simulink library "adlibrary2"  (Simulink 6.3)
undefined symbols (not defined in the file or in its folder): ad_get_simulink_period, adlibrary2, ADM, blue, Boolean, C, c7c04a0c, CIN, constant, DDRII, gcbh, II, no_bitstream, P, SRAM, SX, VER_STRING_GOES_HERE, white, xlBlockLoadCallback, XP, XRC
libraries: xbsIndex_r4 x299, adlibrary2 x7, adlibrary2_d2sram_0 x5, adlibrary2_ddr_xpi0 x4, adlibrary2_ddr_xpl x3, adlibrary2_xpl32 x1, adlibrary2_xpl64 x1, adlibrary2_zbt64 x1, adlibrary2_zbt4_0 x1, adlibrary2_zbt4_1 x1, adlibrary2_zbt4_2 x1, adlibrary2_zbt4_3 x1
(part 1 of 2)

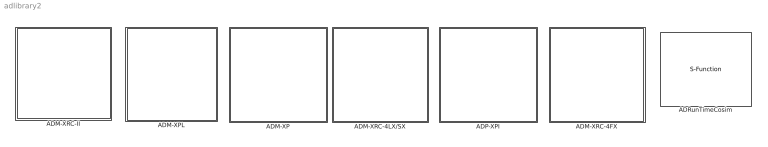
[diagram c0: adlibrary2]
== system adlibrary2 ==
  ADM-XP : Subsystem
  ADM-XPL : Subsystem
  ADM-XRC-4FX : Subsystem  AncestorBlock=adlibrary2/ADM-XRC-4LX//SX
  ADM-XRC-4LX/SX : Subsystem  AncestorBlock=adlibrary2/ADM-XRC-II
  ADM-XRC-II : Subsystem
  ADP-XPI : Subsystem
  ADRunTimeCosim : S-Function  FunctionName=adcosim  Parameters='',index,bitstream,freq,single_step,shared  mask{index=0, bitstream=no_bitstream, freq=50, single_step=off, shared=None}
      mask prompts: index "Card Index"; freq "Clock Frequency"; single_step "Single Step"; shared "Share Access"

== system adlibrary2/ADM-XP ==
  DDR SDRAM 0 : Subsystem  mask{memsize=1}
      mask prompts: memsize "Simulation RAM Size (Mb)"
  DDR SDRAM 1 : Subsystem  mask{memsize=1}
      mask prompts: memsize "Simulation RAM Size (Mb)"
  DDRII SRAM 0 : Subsystem  mask{rate=1}
      mask prompts: rate "Simulink Clock Period"
  DDRII SRAM 1 : Subsystem  AncestorBlock=adlibrary2/ADM-XP/DDRII SRAM 0  mask{rate=1}
      mask prompts: rate "Simulink Clock Period"
  DDRII SRAM 2 : Subsystem  mask{rate=1}
      mask prompts: rate "Simulink Clock Period"
  DDRII SRAM 3 : Subsystem  mask{rate=1}
      mask prompts: rate "Simulink Clock Period"
  XPL 32 Bit Interface : adlibrary2/ADM-XPL/XPL 32 Bit Interface  program='load myprogram.txt'  clock_ratio=1.5  sstep_clk_sel_default=0
  XPL 64 Bit Interface : adlibrary2/ADM-XPL/XPL 64 Bit Interface  program='load myprogram.txt'  clock_ratio=1.5  sstep_clk_sel_default=0

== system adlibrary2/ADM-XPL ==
  DDR SDRAM : Subsystem  mask{memsize=1}
      mask prompts: memsize "Simulation RAM Size (Mb)"
  XPL 32 Bit Interface : Subsystem  mask{program='load myprogram.txt', clock_ratio=1.5, sstep_clk_sel_default=0}
      mask prompts: program "Local Bus Script Program"; clock_ratio "Clock Ratio"
  XPL 64 Bit Interface : Subsystem  mask{program='load myprogram.txt', clock_ratio=1.5, sstep_clk_sel_default=0}
      mask prompts: program "Local Bus Script Program"; clock_ratio "Clock Ratio"
  ZBT SRAM 64 : Subsystem  mask{rate=1}
      mask prompts: rate "Simulink Clock Period"

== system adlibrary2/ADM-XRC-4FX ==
  XPL 32 Bit Interface : adlibrary2/ADM-XPL/XPL 32 Bit Interface  program='load myprogram.txt'  clock_ratio=1.5  sstep_clk_sel_default=0
  XPL 64 Bit Interface : adlibrary2/ADM-XPL/XPL 64 Bit Interface  program='load myprogram.txt'  clock_ratio=1.5  sstep_clk_sel_default=0

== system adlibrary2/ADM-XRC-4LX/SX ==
  PLX 32 Bit Interface : adlibrary2/ADM-XRC-II/PLX 32 Bit Interface  program='load myprogram.txt'  clock_ratio=1.5  sstep_clk_sel_default=0
  ZBT SRAM 0 : Subsystem
  ZBT SRAM 1 : Subsystem
  ZBT SRAM 2 : Subsystem
  ZBT SRAM 3 : Subsystem
  ZBT SRAM 4 : Subsystem
  ZBT SRAM 5 : Subsystem

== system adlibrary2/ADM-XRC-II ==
  PLX 32 Bit Interface : Subsystem  mask{program='load myprogram.txt', clock_ratio=1.5, sstep_clk_sel_default=0}
      mask prompts: program "Local Bus Script Program"; clock_ratio "Clock Ratio"
  "XRM DDR SDRAM " : Subsystem  mask{memsize=1}
      mask prompts: memsize "Simulation RAM Size (Mb)"
  ZBT SRAM 0 : Subsystem  mask{rate=1}
      mask prompts: rate "Simulink Clock Period"
  ZBT SRAM 1 : Subsystem  mask{rate=1}
      mask prompts: rate "Simulink Clock Period"
  ZBT SRAM 2 : Subsystem  mask{rate=1}
      mask prompts: rate "Simulink Clock Period"
  ZBT SRAM 3 : Subsystem  mask{rate=1}
      mask prompts: rate "Simulink Clock Period"
  ZBT SRAM 4 : Subsystem  mask{rate=1}
      mask prompts: rate "Simulink Clock Period"
  ZBT SRAM 5 : Subsystem  mask{rate=1}
      mask prompts: rate "Simulink Clock Period:"

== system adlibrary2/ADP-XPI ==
  DDR SDRAM 0 : Subsystem  mask{memsize=1}
      mask prompts: memsize "Simulation RAM Size (Mb)"
  DDR SDRAM 1 : Subsystem  mask{memsize=1}
      mask prompts: memsize "Simulation RAM Size (Mb)"
  DDR SDRAM 2 : Subsystem  mask{memsize=1}
      mask prompts: memsize "Simulation RAM Size (Mb)"
  DDR SDRAM 3 : Subsystem  mask{memsize=1}
      mask prompts: memsize "Simulation RAM Size (Mb)"
  DDRII SRAM 0 : Subsystem
  XPL 32 Bit Interface : adlibrary2/ADM-XPL/XPL 32 Bit Interface  program='load myprogram.txt'  clock_ratio=1.5  sstep_clk_sel_default=0
  XPL 64 Bit Interface : adlibrary2/ADM-XPL/XPL 64 Bit Interface  program='load myprogram.txt'  clock_ratio=1.5  sstep_clk_sel_default=0

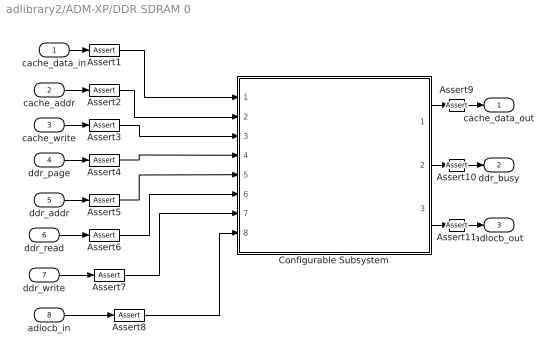
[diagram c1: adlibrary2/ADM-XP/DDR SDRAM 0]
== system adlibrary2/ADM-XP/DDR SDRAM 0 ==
  cache_data_in : Inport
  cache_addr : Inport  Port=2
  cache_write : Inport  Port=3
  ddr_page : Inport  Port=4
  ddr_addr : Inport  Port=5
  ddr_read : Inport  Port=6
  ddr_write : Inport  Port=7
  adlocb_in : Inport  Port=8
  Assert{1..11} (11 alike) : xbsIndex_r4/Assert  assert_type=off  type_source=Explicitly  arith_type="Signed  (2's comp)"  n_bits=16  bin_pt=14  assert_rate=on  rate_source=Explicitly  period=ad_get_simulink_period  output_port=on  block_type=assert
  Configurable Subsystem : Subsystem  Tag=configX  BlockChoice=DDR SDRAM 32bit Simulation  mask{memsize=memsize}
      mask prompts: memsize "Simulation Ram Size (Mb)"
  cache_data_out : Outport
  ddr_busy : Outport  Port=2
  adlocb_out : Outport  Port=3
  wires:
  Configurable Subsystem/3(adlocb_out) -> Assert11/1
  Configurable Subsystem/2(ddr_busy) -> Assert10/1
  Configurable Subsystem/1(cache_data_out) -> Assert9/1
  cache_data_in/1 -> Assert1/1
  cache_addr/1 -> Assert2/1
  cache_write/1 -> Assert3/1
  ddr_page/1 -> Assert4/1
  ddr_addr/1 -> Assert5/1
  ddr_read/1 -> Assert6/1
  ddr_write/1 -> Assert7/1
  adlocb_in/1 -> Assert8/1
  Assert1/1 -> Configurable Subsystem/1(cache_data_in)
  Assert2/1 -> Configurable Subsystem/2(cache_addr)
  Assert3/1 -> Configurable Subsystem/3(cache_write)
  Assert4/1 -> Configurable Subsystem/4(ddr_page)
  Assert5/1 -> Configurable Subsystem/5(ddr_addr)
  Assert6/1 -> Configurable Subsystem/6(ddr_read)
  Assert7/1 -> Configurable Subsystem/7(ddr_write)
  Assert8/1 -> Configurable Subsystem/8(adlocb_in)
  Assert9/1 -> cache_data_out/1
  Assert10/1 -> ddr_busy/1
  Assert11/1 -> adlocb_out/1

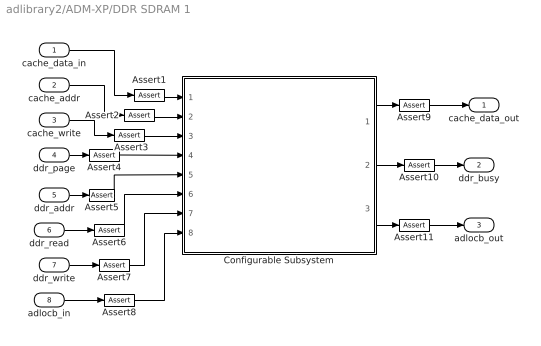
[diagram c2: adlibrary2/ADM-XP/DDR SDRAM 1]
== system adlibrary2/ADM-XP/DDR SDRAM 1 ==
  cache_data_in : Inport
  cache_addr : Inport  Port=2
  cache_write : Inport  Port=3
  ddr_page : Inport  Port=4
  ddr_addr : Inport  Port=5
  ddr_read : Inport  Port=6
  ddr_write : Inport  Port=7
  adlocb_in : Inport  Port=8
  Assert{1..11} (11 alike) : xbsIndex_r4/Assert  assert_type=off  type_source=Explicitly  arith_type="Signed  (2's comp)"  n_bits=16  bin_pt=14  assert_rate=on  rate_source=Explicitly  period=ad_get_simulink_period  output_port=on  block_type=assert
  Configurable Subsystem : Subsystem  Tag=configX  BlockChoice=DDR SDRAM 32bit Simulation  mask{memsize=memsize}
      mask prompts: memsize "Simulation Ram Size (Mb)"
  cache_data_out : Outport
  ddr_busy : Outport  Port=2
  adlocb_out : Outport  Port=3
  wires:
  Configurable Subsystem/3(adlocb_out) -> Assert11/1
  Configurable Subsystem/2(ddr_busy) -> Assert10/1
  Configurable Subsystem/1(cache_data_out) -> Assert9/1
  cache_data_in/1 -> Assert1/1
  cache_addr/1 -> Assert2/1
  cache_write/1 -> Assert3/1
  ddr_page/1 -> Assert4/1
  ddr_addr/1 -> Assert5/1
  ddr_read/1 -> Assert6/1
  ddr_write/1 -> Assert7/1
  adlocb_in/1 -> Assert8/1
  Assert1/1 -> Configurable Subsystem/1(cache_data_in)
  Assert2/1 -> Configurable Subsystem/2(cache_addr)
  Assert3/1 -> Configurable Subsystem/3(cache_write)
  Assert4/1 -> Configurable Subsystem/4(ddr_page)
  Assert5/1 -> Configurable Subsystem/5(ddr_addr)
  Assert6/1 -> Configurable Subsystem/6(ddr_read)
  Assert7/1 -> Configurable Subsystem/7(ddr_write)
  Assert8/1 -> Configurable Subsystem/8(adlocb_in)
  Assert9/1 -> cache_data_out/1
  Assert10/1 -> ddr_busy/1
  Assert11/1 -> adlocb_out/1

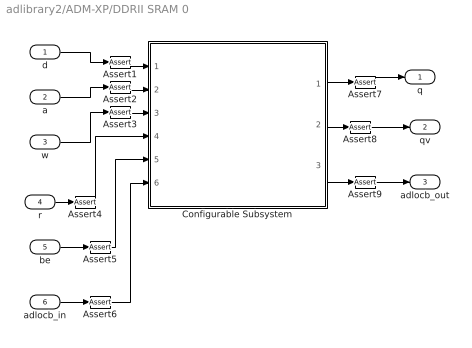
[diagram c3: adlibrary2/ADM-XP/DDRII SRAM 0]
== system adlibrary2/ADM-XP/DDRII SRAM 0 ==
  d : Inport
  a : Inport  Port=2
  w : Inport  Port=3
  r : Inport  Port=4
  be : Inport  Port=5
  adlocb_in : Inport  Port=6
  Assert{1..9} (9 alike) : xbsIndex_r4/Assert  assert_type=off  type_source=Explicitly  arith_type="Signed  (2's comp)"  n_bits=16  bin_pt=14  assert_rate=on  rate_source=Explicitly  period=ad_get_simulink_period  output_port=on  block_type=assert
  Configurable Subsystem : Subsystem  Tag=configX  BlockChoice=DDRII SRAM Simulation
  q : Outport
  qv : Outport  Port=2
  adlocb_out : Outport  Port=3
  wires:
  Configurable Subsystem/1(q) -> Assert7/1
  d/1 -> Assert1/1
  a/1 -> Assert2/1
  w/1 -> Assert3/1
  r/1 -> Assert4/1
  be/1 -> Assert5/1
  adlocb_in/1 -> Assert6/1
  Configurable Subsystem/3(adlocb_out) -> Assert9/1
  Configurable Subsystem/2(qv) -> Assert8/1
  Assert1/1 -> Configurable Subsystem/1(d)
  Assert2/1 -> Configurable Subsystem/2(a)
  Assert3/1 -> Configurable Subsystem/3(w)
  Assert4/1 -> Configurable Subsystem/4(r)
  Assert5/1 -> Configurable Subsystem/5(be)
  Assert6/1 -> Configurable Subsystem/6(adlocb_in)
  Assert7/1 -> q/1
  Assert8/1 -> qv/1
  Assert9/1 -> adlocb_out/1

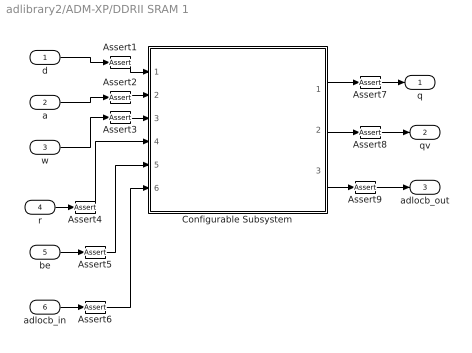
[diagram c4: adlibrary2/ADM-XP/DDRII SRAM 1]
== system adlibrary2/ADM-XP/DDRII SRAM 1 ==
  d : Inport
  a : Inport  Port=2
  w : Inport  Port=3
  r : Inport  Port=4
  be : Inport  Port=5
  adlocb_in : Inport  Port=6
  Assert{1..9} (9 alike) : xbsIndex_r4/Assert  assert_type=off  type_source=Explicitly  arith_type="Signed  (2's comp)"  n_bits=16  bin_pt=14  assert_rate=on  rate_source=Explicitly  period=ad_get_simulink_period  output_port=on  block_type=assert
  Configurable Subsystem : Subsystem  Tag=configX  BlockChoice=DDRII SRAM Simulation
  q : Outport
  qv : Outport  Port=2
  adlocb_out : Outport  Port=3
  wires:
  Configurable Subsystem/1(q) -> Assert7/1
  d/1 -> Assert1/1
  a/1 -> Assert2/1
  w/1 -> Assert3/1
  r/1 -> Assert4/1
  be/1 -> Assert5/1
  adlocb_in/1 -> Assert6/1
  Configurable Subsystem/3(adlocb_out) -> Assert9/1
  Configurable Subsystem/2(qv) -> Assert8/1
  Assert1/1 -> Configurable Subsystem/1(d)
  Assert2/1 -> Configurable Subsystem/2(a)
  Assert3/1 -> Configurable Subsystem/3(w)
  Assert4/1 -> Configurable Subsystem/4(r)
  Assert5/1 -> Configurable Subsystem/5(be)
  Assert6/1 -> Configurable Subsystem/6(adlocb_in)
  Assert7/1 -> q/1
  Assert8/1 -> qv/1
  Assert9/1 -> adlocb_out/1

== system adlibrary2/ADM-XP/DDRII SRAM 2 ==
  d : Inport
  a : Inport  Port=2
  w : Inport  Port=3
  r : Inport  Port=4
  be : Inport  Port=5
  adlocb_in : Inport  Port=6
  Assert{1..9} (9 alike) : xbsIndex_r4/Assert  assert_type=off  type_source=Explicitly  arith_type="Signed  (2's comp)"  n_bits=16  bin_pt=14  assert_rate=on  rate_source=Explicitly  period=ad_get_simulink_period  output_port=on  block_type=assert
  Configurable Subsystem : Subsystem  Tag=configX  BlockChoice=DDRII SRAM Simulation
  q : Outport
  qv : Outport  Port=2
  adlocb_out : Outport  Port=3
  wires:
  Configurable Subsystem/2(qv) -> Assert8/1
  Configurable Subsystem/3(adlocb_out) -> Assert9/1
  adlocb_in/1 -> Assert6/1
  be/1 -> Assert5/1
  r/1 -> Assert4/1
  w/1 -> Assert3/1
  a/1 -> Assert2/1
  d/1 -> Assert1/1
  Configurable Subsystem/1(q) -> Assert7/1
  Assert7/1 -> q/1
  Assert8/1 -> qv/1
  Assert9/1 -> adlocb_out/1
  Assert1/1 -> Configurable Subsystem/1(d)
  Assert2/1 -> Configurable Subsystem/2(a)
  Assert3/1 -> Configurable Subsystem/3(w)
  Assert4/1 -> Configurable Subsystem/4(r)
  Assert5/1 -> Configurable Subsystem/5(be)
  Assert6/1 -> Configurable Subsystem/6(adlocb_in)

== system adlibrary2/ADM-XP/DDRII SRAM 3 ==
  d : Inport
  a : Inport  Port=2
  w : Inport  Port=3
  r : Inport  Port=4
  be : Inport  Port=5
  adlocb_in : Inport  Port=6
  Assert{1..9} (9 alike) : xbsIndex_r4/Assert  assert_type=off  type_source=Explicitly  arith_type="Signed  (2's comp)"  n_bits=16  bin_pt=14  assert_rate=on  rate_source=Explicitly  period=ad_get_simulink_period  output_port=on  block_type=assert
  Configurable Subsystem : Subsystem  Tag=configX  BlockChoice=DDRII SRAM Simulation
  q : Outport
  qv : Outport  Port=2
  adlocb_out : Outport  Port=3
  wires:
  Configurable Subsystem/2(qv) -> Assert8/1
  Configurable Subsystem/3(adlocb_out) -> Assert9/1
  adlocb_in/1 -> Assert6/1
  be/1 -> Assert5/1
  r/1 -> Assert4/1
  w/1 -> Assert3/1
  a/1 -> Assert2/1
  d/1 -> Assert1/1
  Configurable Subsystem/1(q) -> Assert7/1
  Assert1/1 -> Configurable Subsystem/1(d)
  Assert2/1 -> Configurable Subsystem/2(a)
  Assert3/1 -> Configurable Subsystem/3(w)
  Assert4/1 -> Configurable Subsystem/4(r)
  Assert5/1 -> Configurable Subsystem/5(be)
  Assert6/1 -> Configurable Subsystem/6(adlocb_in)
  Assert7/1 -> q/1
  Assert8/1 -> qv/1
  Assert9/1 -> adlocb_out/1

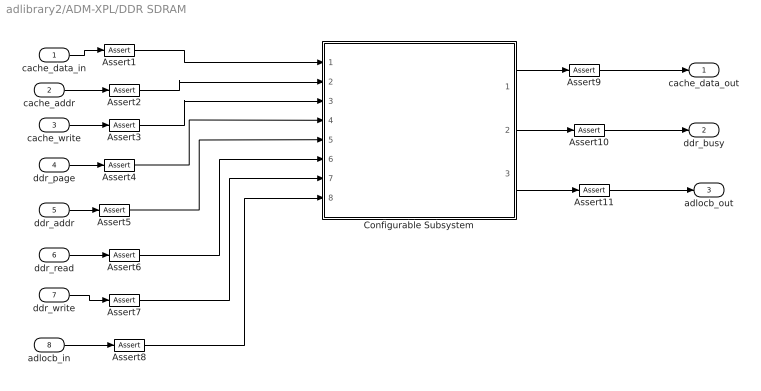
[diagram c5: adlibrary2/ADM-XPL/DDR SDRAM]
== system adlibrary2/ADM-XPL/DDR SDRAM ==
  cache_data_in : Inport
  cache_addr : Inport  Port=2
  cache_write : Inport  Port=3
  ddr_page : Inport  Port=4
  ddr_addr : Inport  Port=5
  ddr_read : Inport  Port=6
  ddr_write : Inport  Port=7
  adlocb_in : Inport  Port=8
  Assert{1..11} (11 alike) : xbsIndex_r4/Assert  assert_type=off  type_source=Explicitly  arith_type="Signed  (2's comp)"  n_bits=16  bin_pt=14  assert_rate=on  rate_source=Explicitly  period=ad_get_simulink_period  output_port=on  block_type=assert
  Configurable Subsystem : Subsystem  Tag=configX  BlockChoice=DDR SDRAM 32bit Simulation  mask{memsize=memsize}
      mask prompts: memsize "Simulation Ram Size (Mb)"
  cache_data_out : Outport
  ddr_busy : Outport  Port=2
  adlocb_out : Outport  Port=3
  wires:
  cache_data_in/1 -> Assert1/1
  cache_addr/1 -> Assert2/1
  cache_write/1 -> Assert3/1
  ddr_page/1 -> Assert4/1
  ddr_addr/1 -> Assert5/1
  ddr_read/1 -> Assert6/1
  ddr_write/1 -> Assert7/1
  adlocb_in/1 -> Assert8/1
  Configurable Subsystem/1(cache_data_out) -> Assert9/1
  Configurable Subsystem/2(ddr_busy) -> Assert10/1
  Configurable Subsystem/3(adlocb_out) -> Assert11/1
  Assert1/1 -> Configurable Subsystem/1(cache_data_in)
  Assert2/1 -> Configurable Subsystem/2(cache_addr)
  Assert3/1 -> Configurable Subsystem/3(cache_write)
  Assert4/1 -> Configurable Subsystem/4(ddr_page)
  Assert5/1 -> Configurable Subsystem/5(ddr_addr)
  Assert6/1 -> Configurable Subsystem/6(ddr_read)
  Assert7/1 -> Configurable Subsystem/7(ddr_write)
  Assert8/1 -> Configurable Subsystem/8(adlocb_in)
  Assert9/1 -> cache_data_out/1
  Assert10/1 -> ddr_busy/1
  Assert11/1 -> adlocb_out/1

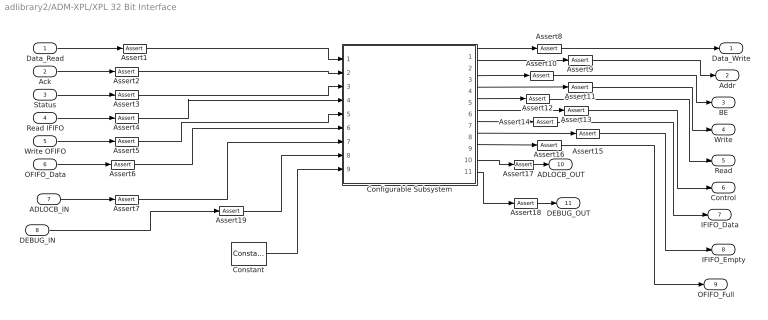
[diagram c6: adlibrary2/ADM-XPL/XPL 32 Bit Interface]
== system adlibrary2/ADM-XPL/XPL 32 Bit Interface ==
  Data_Read : Inport
  Ack : Inport  Port=2
  Status : Inport  Port=3
  Read IFIFO : Inport  Port=4
  Write OFIFO : Inport  Port=5
  OFIFO_Data : Inport  Port=6
  ADLOCB_IN : Inport  Port=7
  DEBUG_IN : Inport  Port=8
  Assert{1..19} (19 alike) : xbsIndex_r4/Assert  assert_type=off  type_source=Explicitly  arith_type="Signed  (2's comp)"  n_bits=16  bin_pt=14  assert_rate=on  rate_source=Explicitly  period=ad_get_simulink_period  output_port=on  block_type=assert
  Configurable Subsystem : Subsystem  Tag=configX  BlockChoice=XPL 32Bit Simulation  mask{program=program, clock_ratio=clock_ratio}
      mask prompts: program "Local Bus Script Program"; clock_ratio "Clock Ratio"
  Constant : xbsIndex_r4/Constant  arith_type=Boolean  const=sstep_clk_sel_default  n_bits=16  bin_pt=14  explicit_period=on  period=ad_get_simulink_period  equ=P=C  opselect=C  inp2=PCIN>>17  opr=+  inp1=P  carry=CIN  dbl_ovrd=off  block_type=constant
  Data_Write : Outport
  Addr : Outport  Port=2
  BE : Outport  Port=3
  Write : Outport  Port=4
  Read : Outport  Port=5
  Control : Outport  Port=6
  IFIFO_Data : Outport  Port=7
  IFIFO_Empty : Outport  Port=8
  OFIFO_Full : Outport  Port=9
  ADLOCB_OUT : Outport  Port=10
  DEBUG_OUT : Outport  Port=11
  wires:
  Status/1 -> Assert3/1
  Ack/1 -> Assert2/1
  Data_Read/1 -> Assert1/1
  Configurable Subsystem/9(OFIFO_Full) -> Assert16/1
  Configurable Subsystem/8(IFIFO_Empty) -> Assert15/1
  Configurable Subsystem/7(IFIFO_Data) -> Assert14/1
  Configurable Subsystem/6(Control) -> Assert13/1
  Configurable Subsystem/5(Read) -> Assert12/1
  Configurable Subsystem/4(Write) -> Assert11/1
  Configurable Subsystem/3(BE) -> Assert10/1
  Configurable Subsystem/1(Data_Write) -> Assert8/1
  Configurable Subsystem/2(Addr) -> Assert9/1
  Read IFIFO/1 -> Assert4/1
  Write OFIFO/1 -> Assert5/1
  OFIFO_Data/1 -> Assert6/1
  ADLOCB_IN/1 -> Assert7/1
  Configurable Subsystem/10(ADLOCB_OUT) -> Assert17/1
  Assert1/1 -> Configurable Subsystem/1(Data_Read)
  Assert2/1 -> Configurable Subsystem/2(Ack)
  Assert3/1 -> Configurable Subsystem/3(Status)
  Assert4/1 -> Configurable Subsystem/4(Read IFIFO)
  Assert8/1 -> Data_Write/1
  Assert9/1 -> Addr/1
  Assert10/1 -> BE/1
  Assert11/1 -> Write/1
  Assert12/1 -> Read/1
  Assert13/1 -> Control/1
  Assert14/1 -> IFIFO_Data/1
  Assert15/1 -> IFIFO_Empty/1
  Assert16/1 -> OFIFO_Full/1
  Assert17/1 -> ADLOCB_OUT/1
  Assert5/1 -> Configurable Subsystem/5(Write OFIFO)
  Assert6/1 -> Configurable Subsystem/6(OFIFO_Data)
  Assert7/1 -> Configurable Subsystem/7(ADLOCB_IN)
  DEBUG_IN/1 -> Assert19/1
  Assert19/1 -> Configurable Subsystem/8(DEBUG_IN)
  Assert18/1 -> DEBUG_OUT/1
  Configurable Subsystem/11(DEBUG_OUT) -> Assert18/1
  Constant/1 -> Configurable Subsystem/9(sstep_clk_sel_default)

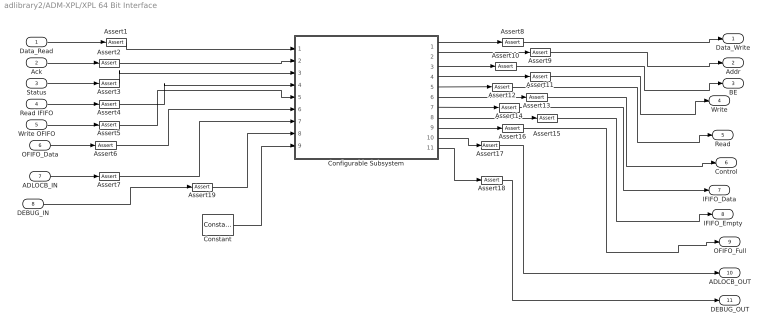
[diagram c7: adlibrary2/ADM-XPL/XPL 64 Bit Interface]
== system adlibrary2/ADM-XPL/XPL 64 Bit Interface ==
  Data_Read : Inport
  Ack : Inport  Port=2
  Status : Inport  Port=3
  Read IFIFO : Inport  Port=4
  Write OFIFO : Inport  Port=5
  OFIFO_Data : Inport  Port=6
  ADLOCB_IN : Inport  Port=7
  DEBUG_IN : Inport  Port=8
  Assert{1..19} (19 alike) : xbsIndex_r4/Assert  assert_type=off  type_source=Explicitly  arith_type="Signed  (2's comp)"  n_bits=16  bin_pt=14  assert_rate=on  rate_source=Explicitly  period=ad_get_simulink_period  output_port=on  block_type=assert
  Configurable Subsystem : Subsystem  Tag=configX  BlockChoice=XPL 64Bit Simulation  mask{program=program, clock_ratio=clock_ratio}
      mask prompts: program "Local Bus Script Program"; clock_ratio "Clock Ratio"
  Constant : xbsIndex_r4/Constant  arith_type=Boolean  const=sstep_clk_sel_default  n_bits=16  bin_pt=14  explicit_period=on  period=ad_get_simulink_period  equ=P=C  opselect=C  inp2=PCIN>>17  opr=+  inp1=P  carry=CIN  dbl_ovrd=off  block_type=constant
  Data_Write : Outport
  Addr : Outport  Port=2
  BE : Outport  Port=3
  Write : Outport  Port=4
  Read : Outport  Port=5
  Control : Outport  Port=6
  IFIFO_Data : Outport  Port=7
  IFIFO_Empty : Outport  Port=8
  OFIFO_Full : Outport  Port=9
  ADLOCB_OUT : Outport  Port=10
  DEBUG_OUT : Outport  Port=11
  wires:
  Status/1 -> Assert3/1
  Ack/1 -> Assert2/1
  Data_Read/1 -> Assert1/1
  Read IFIFO/1 -> Assert4/1
  Write OFIFO/1 -> Assert5/1
  OFIFO_Data/1 -> Assert6/1
  ADLOCB_IN/1 -> Assert7/1
  Assert1/1 -> Configurable Subsystem/1(Data_Read)
  Assert2/1 -> Configurable Subsystem/2(Ack)
  Assert3/1 -> Configurable Subsystem/3(Status)
  Assert4/1 -> Configurable Subsystem/4(Read IFIFO)
  Assert5/1 -> Configurable Subsystem/5(Write OFIFO)
  Assert6/1 -> Configurable Subsystem/6(OFIFO_Data)
  Assert7/1 -> Configurable Subsystem/7(ADLOCB_IN)
  DEBUG_IN/1 -> Assert19/1
  Assert19/1 -> Configurable Subsystem/8(DEBUG_IN)
  Constant/1 -> Configurable Subsystem/9(sstep_clk_sel_default)
  Configurable Subsystem/9(OFIFO_Full) -> Assert16/1
  Configurable Subsystem/8(IFIFO_Empty) -> Assert15/1
  Configurable Subsystem/7(IFIFO_Data) -> Assert14/1
  Configurable Subsystem/6(Control) -> Assert13/1
  Configurable Subsystem/5(Read) -> Assert12/1
  Configurable Subsystem/4(Write) -> Assert11/1
  Configurable Subsystem/3(BE) -> Assert10/1
  Configurable Subsystem/1(Data_Write) -> Assert8/1
  Configurable Subsystem/2(Addr) -> Assert9/1
  Configurable Subsystem/10(ADLOCB_OUT) -> Assert17/1
  Assert8/1 -> Data_Write/1
  Assert9/1 -> Addr/1
  Assert10/1 -> BE/1
  Assert11/1 -> Write/1
  Assert12/1 -> Read/1
  Assert13/1 -> Control/1
  Assert14/1 -> IFIFO_Data/1
  Assert15/1 -> IFIFO_Empty/1
  Assert16/1 -> OFIFO_Full/1
  Assert17/1 -> ADLOCB_OUT/1
  Assert18/1 -> DEBUG_OUT/1
  Configurable Subsystem/11(DEBUG_OUT) -> Assert18/1

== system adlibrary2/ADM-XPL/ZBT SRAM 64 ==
  d : Inport
  a : Inport  Port=2
  w : Inport  Port=3
  r : Inport  Port=4
  be : Inport  Port=5
  adlocb_in : Inport  Port=6
  Assert{1..9} (9 alike) : xbsIndex_r4/Assert  assert_type=off  type_source=Explicitly  arith_type="Signed  (2's comp)"  n_bits=16  bin_pt=14  assert_rate=on  rate_source=Explicitly  period=ad_get_simulink_period  output_port=on  block_type=assert
  Configurable Subsystem : Subsystem  Tag=configX  BlockChoice=ZBT SRAM 64bit Simulation
  q : Outport
  qv : Outport  Port=2
  adlocb_out : Outport  Port=3
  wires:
  d/1 -> Assert1/1
  a/1 -> Assert2/1
  w/1 -> Assert3/1
  r/1 -> Assert4/1
  be/1 -> Assert5/1
  adlocb_in/1 -> Assert6/1
  Configurable Subsystem/1(q) -> Assert7/1
  Configurable Subsystem/2(qv) -> Assert8/1
  Configurable Subsystem/3(adlocb_out) -> Assert9/1
  Assert1/1 -> Configurable Subsystem/1(d)
  Assert2/1 -> Configurable Subsystem/2(a)
  Assert3/1 -> Configurable Subsystem/3(w)
  Assert4/1 -> Configurable Subsystem/4(r)
  Assert5/1 -> Configurable Subsystem/5(be)
  Assert6/1 -> Configurable Subsystem/6(adlocb_in)
  Assert7/1 -> q/1
  Assert8/1 -> qv/1
  Assert9/1 -> adlocb_out/1

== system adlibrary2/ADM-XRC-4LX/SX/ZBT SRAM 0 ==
  d : Inport
  a : Inport  Port=2
  w : Inport  Port=3
  r : Inport  Port=4
  be : Inport  Port=5
  adlocb_in : Inport  Port=6
  Assert{1..9} (9 alike) : xbsIndex_r4/Assert  assert_type=off  type_source=Explicitly  arith_type="Signed  (2's comp)"  n_bits=16  bin_pt=14  assert_rate=on  rate_source=Explicitly  period=ad_get_simulink_period  output_port=on  block_type=assert
  Configurable Subsystem : Subsystem  Tag=configX  BlockChoice=ZBT SRAM 32Bit Simulation
  q : Outport
  qv : Outport  Port=2
  adlocb_out : Outport  Port=3
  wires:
  Configurable Subsystem/3(adlocb_out) -> Assert9/1
  Configurable Subsystem/2(qv) -> Assert8/1
  Configurable Subsystem/1(q) -> Assert7/1
  adlocb_in/1 -> Assert6/1
  be/1 -> Assert5/1
  r/1 -> Assert4/1
  w/1 -> Assert3/1
  a/1 -> Assert2/1
  d/1 -> Assert1/1
  Assert1/1 -> Configurable Subsystem/1(d)
  Assert2/1 -> Configurable Subsystem/2(a)
  Assert3/1 -> Configurable Subsystem/3(w)
  Assert4/1 -> Configurable Subsystem/4(r)
  Assert5/1 -> Configurable Subsystem/5(be)
  Assert6/1 -> Configurable Subsystem/6(adlocb_in)
  Assert7/1 -> q/1
  Assert8/1 -> qv/1
  Assert9/1 -> adlocb_out/1

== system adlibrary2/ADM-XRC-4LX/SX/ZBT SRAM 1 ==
  d : Inport
  a : Inport  Port=2
  w : Inport  Port=3
  r : Inport  Port=4
  be : Inport  Port=5
  adlocb_in : Inport  Port=6
  Assert{1..9} (9 alike) : xbsIndex_r4/Assert  assert_type=off  type_source=Explicitly  arith_type="Signed  (2's comp)"  n_bits=16  bin_pt=14  assert_rate=on  rate_source=Explicitly  period=ad_get_simulink_period  output_port=on  block_type=assert
  Configurable Subsystem : Subsystem  Tag=configX  BlockChoice=ZBT SRAM 32Bit Simulation
  q : Outport
  qv : Outport  Port=2
  adlocb_out : Outport  Port=3
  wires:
  d/1 -> Assert1/1
  a/1 -> Assert2/1
  w/1 -> Assert3/1
  r/1 -> Assert4/1
  be/1 -> Assert5/1
  adlocb_in/1 -> Assert6/1
  Configurable Subsystem/1(q) -> Assert7/1
  Configurable Subsystem/2(qv) -> Assert8/1
  Configurable Subsystem/3(adlocb_out) -> Assert9/1
  Assert1/1 -> Configurable Subsystem/1(d)
  Assert2/1 -> Configurable Subsystem/2(a)
  Assert3/1 -> Configurable Subsystem/3(w)
  Assert4/1 -> Configurable Subsystem/4(r)
  Assert5/1 -> Configurable Subsystem/5(be)
  Assert6/1 -> Configurable Subsystem/6(adlocb_in)
  Assert7/1 -> q/1
  Assert8/1 -> qv/1
  Assert9/1 -> adlocb_out/1

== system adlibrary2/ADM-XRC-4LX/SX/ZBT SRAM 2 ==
  d : Inport
  a : Inport  Port=2
  w : Inport  Port=3
  r : Inport  Port=4
  be : Inport  Port=5
  adlocb_in : Inport  Port=6
  Assert{1..9} (9 alike) : xbsIndex_r4/Assert  assert_type=off  type_source=Explicitly  arith_type="Signed  (2's comp)"  n_bits=16  bin_pt=14  assert_rate=on  rate_source=Explicitly  period=ad_get_simulink_period  output_port=on  block_type=assert
  Configurable Subsystem : Subsystem  Tag=configX  BlockChoice=ZBT SRAM 32Bit Simulation
  q : Outport
  qv : Outport  Port=2
  adlocb_out : Outport  Port=3
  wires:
  d/1 -> Assert1/1
  a/1 -> Assert2/1
  w/1 -> Assert3/1
  r/1 -> Assert4/1
  be/1 -> Assert5/1
  adlocb_in/1 -> Assert6/1
  Configurable Subsystem/1(q) -> Assert8/1
  Configurable Subsystem/2(qv) -> Assert9/1
  Configurable Subsystem/3(adlocb_out) -> Assert7/1
  Assert1/1 -> Configurable Subsystem/1(d)
  Assert2/1 -> Configurable Subsystem/2(a)
  Assert3/1 -> Configurable Subsystem/3(w)
  Assert4/1 -> Configurable Subsystem/4(r)
  Assert5/1 -> Configurable Subsystem/5(be)
  Assert6/1 -> Configurable Subsystem/6(adlocb_in)
  Assert7/1 -> adlocb_out/1
  Assert8/1 -> q/1
  Assert9/1 -> qv/1

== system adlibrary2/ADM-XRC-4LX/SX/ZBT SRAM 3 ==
  d : Inport
  a : Inport  Port=2
  w : Inport  Port=3
  r : Inport  Port=4
  be : Inport  Port=5
  adlocb_in : Inport  Port=6
  Assert{1..9} (9 alike) : xbsIndex_r4/Assert  assert_type=off  type_source=Explicitly  arith_type="Signed  (2's comp)"  n_bits=16  bin_pt=14  assert_rate=on  rate_source=Explicitly  period=ad_get_simulink_period  output_port=on  block_type=assert
  Configurable Subsystem : Subsystem  Tag=configX  BlockChoice=ZBT SRAM 32Bit Simulation
  q : Outport
  qv : Outport  Port=2
  adlocb_out : Outport  Port=3
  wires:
  d/1 -> Assert1/1
  a/1 -> Assert2/1
  w/1 -> Assert3/1
  r/1 -> Assert4/1
  be/1 -> Assert5/1
  adlocb_in/1 -> Assert6/1
  Configurable Subsystem/1(q) -> Assert7/1
  Configurable Subsystem/2(qv) -> Assert8/1
  Configurable Subsystem/3(adlocb_out) -> Assert9/1
  Assert1/1 -> Configurable Subsystem/1(d)
  Assert2/1 -> Configurable Subsystem/2(a)
  Assert3/1 -> Configurable Subsystem/3(w)
  Assert4/1 -> Configurable Subsystem/4(r)
  Assert5/1 -> Configurable Subsystem/5(be)
  Assert6/1 -> Configurable Subsystem/6(adlocb_in)
  Assert7/1 -> q/1
  Assert8/1 -> qv/1
  Assert9/1 -> adlocb_out/1

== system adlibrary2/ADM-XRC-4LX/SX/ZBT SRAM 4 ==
  d : Inport
  a : Inport  Port=2
  w : Inport  Port=3
  r : Inport  Port=4
  be : Inport  Port=5
  adlocb_in : Inport  Port=6
  Assert{1..9} (9 alike) : xbsIndex_r4/Assert  assert_type=off  type_source=Explicitly  arith_type="Signed  (2's comp)"  n_bits=16  bin_pt=14  assert_rate=on  rate_source=Explicitly  period=ad_get_simulink_period  output_port=on  block_type=assert
  Configurable Subsystem : Subsystem  Tag=configX  BlockChoice=ZBT SRAM 32Bit Simulation
  q : Outport
  qv : Outport  Port=2
  adlocb_out : Outport  Port=3
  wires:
  d/1 -> Assert1/1
  a/1 -> Assert2/1
  w/1 -> Assert3/1
  r/1 -> Assert4/1
  be/1 -> Assert5/1
  adlocb_in/1 -> Assert6/1
  Configurable Subsystem/1(q) -> Assert7/1
  Configurable Subsystem/2(qv) -> Assert8/1
  Configurable Subsystem/3(adlocb_out) -> Assert9/1
  Assert1/1 -> Configurable Subsystem/1(d)
  Assert2/1 -> Configurable Subsystem/2(a)
  Assert3/1 -> Configurable Subsystem/3(w)
  Assert4/1 -> Configurable Subsystem/4(r)
  Assert5/1 -> Configurable Subsystem/5(be)
  Assert6/1 -> Configurable Subsystem/6(adlocb_in)
  Assert7/1 -> q/1
  Assert8/1 -> qv/1
  Assert9/1 -> adlocb_out/1

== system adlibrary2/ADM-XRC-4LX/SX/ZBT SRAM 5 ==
  d : Inport
  a : Inport  Port=2
  w : Inport  Port=3
  r : Inport  Port=4
  be : Inport  Port=5
  adlocb_in : Inport  Port=6
  Assert{1..9} (9 alike) : xbsIndex_r4/Assert  assert_type=off  type_source=Explicitly  arith_type="Signed  (2's comp)"  n_bits=16  bin_pt=14  assert_rate=on  rate_source=Explicitly  period=ad_get_simulink_period  output_port=on  block_type=assert
  Configurable Subsystem : Subsystem  Tag=configX  BlockChoice=ZBT SRAM 32Bit Simulation
  q : Outport
  qv : Outport  Port=2
  adlocb_out : Outport  Port=3
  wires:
  d/1 -> Assert1/1
  a/1 -> Assert2/1
  w/1 -> Assert3/1
  r/1 -> Assert4/1
  be/1 -> Assert5/1
  adlocb_in/1 -> Assert6/1
  Configurable Subsystem/1(q) -> Assert7/1
  Configurable Subsystem/2(qv) -> Assert8/1
  Configurable Subsystem/3(adlocb_out) -> Assert9/1
  Assert1/1 -> Configurable Subsystem/1(d)
  Assert2/1 -> Configurable Subsystem/2(a)
  Assert3/1 -> Configurable Subsystem/3(w)
  Assert4/1 -> Configurable Subsystem/4(r)
  Assert5/1 -> Configurable Subsystem/5(be)
  Assert6/1 -> Configurable Subsystem/6(adlocb_in)
  Assert7/1 -> q/1
  Assert8/1 -> qv/1
  Assert9/1 -> adlocb_out/1

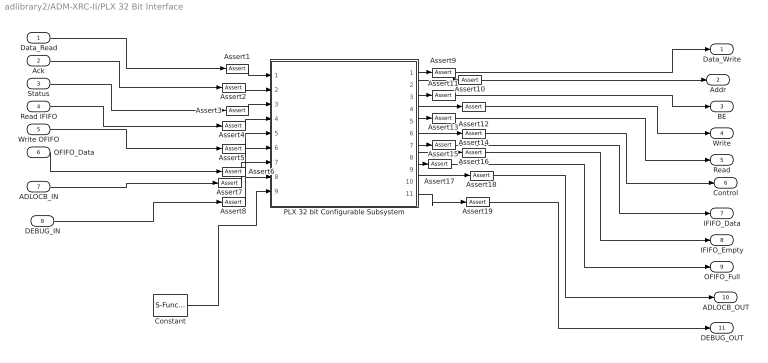
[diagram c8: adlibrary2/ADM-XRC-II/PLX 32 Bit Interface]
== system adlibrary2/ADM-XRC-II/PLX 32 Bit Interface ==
  Data_Read : Inport
  Ack : Inport  Port=2
  Status : Inport  Port=3
  Read IFIFO : Inport  Port=4
  Write OFIFO : Inport  Port=5
  OFIFO_Data : Inport  Port=6
  ADLOCB_IN : Inport  Port=7
  DEBUG_IN : Inport  Port=8
  Assert{1..19} (19 alike) : xbsIndex_r4/Assert  assert_type=off  type_source=Explicitly  arith_type="Signed  (2's comp)"  n_bits=16  bin_pt=14  assert_rate=on  rate_source=Explicitly  period=ad_get_simulink_period  output_port=on  block_type=assert
  Constant : S-Function  AncestorBlock=xbsIndex_r4/Constant  LoadFcn=xlBlockLoadCallback(gcbh);  FunctionName=sysgen  Parameters=ptable_  mask(Xilinx Constant Block Block){arith_type=Boolean, arith_type_sgadvanced=, const=sstep_clk_sel_default, n_bits=16, bin_pt=14, explicit_period=on, explicit_period_sgadvanced=, period=ad_get_simulink_period, equ=P=C, opselect=C, opselect_sgadvanced=, inp2=PCIN>>17, inp2_sgadvanced=, opr=+, opr_sgadvanced=, inp1=P, inp1_sgadvanced=, carry=CIN, carry_sgadvanced=, dbl_ovrd=off, dbl_ovrd_sgadvanced=, block_version=VER_STRING_GOES_HERE, has_advanced_control=0, sggui_pos=-1,-1,-1,-1, block_type=constant, sg_icon_stat=45,30,0,1,white,blue,0,c7c04a0c, sg_mask_display=fprintf('','COMMENT: begin icon graphics '); patch([0 45 45 0 ],[0 0 30 30 ],[0.77 0.82 0.91]); patch([15 10 17 10 15 23 25 27 35 28 22 17 23 17 22 28 35 27 25 23 15 ],[3 8 15 22 27 27 25 27 27 20 26 21 15 9 4 10 3 3 5 3 3 ],[0.98 0.96 0.92]); plot([0 0 45 45 0 ],[0 30 30 0 0 ]); fprintf('','COMMENT: end icon graphics');  fprintf('','COMMENT: begin icon text '); color('black');port_label('output',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, sg_list_contents=}
      mask prompts: arith_type "Type"; const "Constant value"; n_bits "Number of bits"; bin_pt "Binary point"; explicit_period "Sampled constant"; period "Sample period"; equ "DSP48 operation"; opselect "Operation select"; inp2 "Z mux"; opr "Operand"; inp1 "YX muxes"; carry "Carry input"; dbl_ovrd "Override with doubles"; block_version ""; has_advanced_control ""; sggui_pos ""; block_type ""; sg_icon_stat ""; sg_mask_display ""; sg_list_contents ""
      mask help: Xilinx Constant Block
      mask init:
      | xlMungeMaskParams;
      | sav_gcbh = gcbh;
      | op = 0;
      | dsp48instr = 0;
      | if (arith_type==1)
      | bool = 1;
      | k= xltodouble(const,1,0,1,2,2);
      | elseif (arith_type == 4) %dsp48
      | dsp48instr = 1;
      | bool = 0;
      | str = equ;
      | n_bits = 11;
      | bin_pt = 0;
      | arith_type = 1;
      | equ = xlbuildEqnString(sav_gcbh);
      | [op, opmode, sub, carryin, carryin_sel] = xlcalcDSP48OpComplete(opselect,inp2,inp1,opr,carry);;
      | %[op,opmode, sub, carryin, carryin_sel] = xlcalcDSP48Op(equ);
      | elseif (arith_type == 3) %unsigned (arith_type of 2 maps to Signed)
      | bool = 0;
      | arith_type=1;
      | end
      | 
      | precision0 = 2;
      | z0 = [n_bits bin_pt arith_type 2 2];
      | explicitClk = explicit_period;
      | 
      | % ----------------------------------------
      | 
      | block_config = 'Sysgen:legacy_block_config:xlconstant';
      | serialized_declarations = '{''const''=>''Double'',''period''=>''Double'',''simulinkPeriod''=>''Double'',''bool''=>''Int'',''dblOvrd''=>''Int'',''dsp48instr''=>''Int'',''explicitClk''=>''Int'',''hasEN''=>''Int'',''hasRST''=>''Int'',''latency''=>''Int'',''n_bits''=>''Int'',''op''=>''Int'',''opselect''=>''Int'',''carry''=>''Int'',''precision#''=>''Int'',''trimVbit''=>''Int'',''useCore''=>''Int'',''z#''=>''IntVector'',''designRoot''=>''String'',''equ''=>''String'',''family''=>''String'',''block_version''=>''String'',''block_config''=>''String'',}';
      | ptable_ = xlblockprep(get_param(gcb, 'MaskWSVariables'));
  PLX 32 bit Configurable Subsystem : Subsystem  Tag=configX  BlockChoice=PLX 32Bit Simulation  mask{program=program, clock_ratio=clock_ratio}
      mask prompts: program "Local Bus Script Program"; clock_ratio "Clock Ratio"
  Data_Write : Outport
  Addr : Outport  Port=2
  BE : Outport  Port=3
  Write : Outport  Port=4
  Read : Outport  Port=5
  Control : Outport  Port=6
  IFIFO_Data : Outport  Port=7
  IFIFO_Empty : Outport  Port=8
  OFIFO_Full : Outport  Port=9
  ADLOCB_OUT : Outport  Port=10
  DEBUG_OUT : Outport  Port=11
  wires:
  PLX 32 bit Configurable Subsystem/1(Data_Write) -> Assert9/1
  PLX 32 bit Configurable Subsystem/2(Addr) -> Assert10/1
  PLX 32 bit Configurable Subsystem/4(Write) -> Assert12/1
  PLX 32 bit Configurable Subsystem/6(Control) -> Assert14/1
  PLX 32 bit Configurable Subsystem/7(IFIFO_Data) -> Assert15/1
  PLX 32 bit Configurable Subsystem/8(IFIFO_Empty) -> Assert16/1
  PLX 32 bit Configurable Subsystem/9(OFIFO_Full) -> Assert17/1
  PLX 32 bit Configurable Subsystem/3(BE) -> Assert11/1
  PLX 32 bit Configurable Subsystem/10(ADLOCB_OUT) -> Assert18/1
  Data_Read/1 -> Assert1/1
  Ack/1 -> Assert2/1
  Status/1 -> Assert3/1
  Read IFIFO/1 -> Assert4/1
  Write OFIFO/1 -> Assert5/1
  OFIFO_Data/1 -> Assert6/1
  ADLOCB_IN/1 -> Assert7/1
  PLX 32 bit Configurable Subsystem/5(Read) -> Assert13/1
  Assert1/1 -> PLX 32 bit Configurable Subsystem/1(Data_Read)
  Assert2/1 -> PLX 32 bit Configurable Subsystem/2(Ack)
  Assert3/1 -> PLX 32 bit Configurable Subsystem/3(Status)
  Assert4/1 -> PLX 32 bit Configurable Subsystem/4(Read IFIFO)
  Assert5/1 -> PLX 32 bit Configurable Subsystem/5(Write OFIFO)
  Assert6/1 -> PLX 32 bit Configurable Subsystem/6(OFIFO_Data)
  Assert7/1 -> PLX 32 bit Configurable Subsystem/7(ADLOCB_IN)
  Assert9/1 -> Data_Write/1
  Assert10/1 -> Addr/1
  Assert11/1 -> BE/1
  Assert12/1 -> Write/1
  Assert13/1 -> Read/1
  Assert14/1 -> Control/1
  Assert15/1 -> IFIFO_Data/1
  Assert16/1 -> IFIFO_Empty/1
  Assert17/1 -> OFIFO_Full/1
  Assert18/1 -> ADLOCB_OUT/1
  DEBUG_IN/1 -> Assert8/1
  PLX 32 bit Configurable Subsystem/11(DEBUG_OUT) -> Assert19/1
  Assert19/1 -> DEBUG_OUT/1
  Assert8/1 -> PLX 32 bit Configurable Subsystem/8(DEBUG_IN)
  Constant/1 -> PLX 32 bit Configurable Subsystem/9(sstep_clk_sel_default)

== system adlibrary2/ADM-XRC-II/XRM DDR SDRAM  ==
  cache_data_in : Inport
  cache_addr : Inport  Port=2
  cache_write : Inport  Port=3
  ddr_page : Inport  Port=4
  ddr_addr : Inport  Port=5
  ddr_read : Inport  Port=6
  ddr_write : Inport  Port=7
  Assert{1..9} (9 alike) : xbsIndex_r4/Assert  assert_type=off  type_source=Explicitly  arith_type="Signed  (2's comp)"  n_bits=16  bin_pt=14  assert_rate=on  rate_source=Explicitly  period=ad_get_simulink_period  output_port=on  block_type=assert
  Configurable Subsystem : Subsystem  Tag=configX  BlockChoice=DDR SDRAM 64bit Simulation
  cache_data_out : Outport
  ddr_busy : Outport  Port=2
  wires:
  cache_data_in/1 -> Assert1/1
  cache_addr/1 -> Assert2/1
  cache_write/1 -> Assert3/1
  ddr_page/1 -> Assert4/1
  ddr_addr/1 -> Assert5/1
  ddr_read/1 -> Assert6/1
  ddr_write/1 -> Assert7/1
  Configurable Subsystem/1(cache_data_out) -> Assert8/1
  Configurable Subsystem/2(ddr_busy) -> Assert9/1
  Assert1/1 -> Configurable Subsystem/1(cache_data_in)
  Assert2/1 -> Configurable Subsystem/2(cache_addr)
  Assert3/1 -> Configurable Subsystem/3(cache_write)
  Assert4/1 -> Configurable Subsystem/4(ddr_page)
  Assert5/1 -> Configurable Subsystem/5(ddr_addr)
  Assert6/1 -> Configurable Subsystem/6(ddr_read)
  Assert7/1 -> Configurable Subsystem/7(ddr_write)
  Assert8/1 -> cache_data_out/1
  Assert9/1 -> ddr_busy/1

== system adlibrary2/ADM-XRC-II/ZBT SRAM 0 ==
  d : Inport
  a : Inport  Port=2
  w : Inport  Port=3
  r : Inport  Port=4
  be : Inport  Port=5
  adlocb_in : Inport  Port=6
  Assert{,1..8} (9 alike) : xbsIndex_r4/Assert  assert_type=off  type_source=Explicitly  arith_type="Signed  (2's comp)"  n_bits=16  bin_pt=14  assert_rate=on  rate_source=Explicitly  period=ad_get_simulink_period  output_port=on  block_type=assert
  Configurable Subsystem : Subsystem  Tag=configX  BlockChoice=ZBT SRAM 32Bit Simulation
  q : Outport
  qv : Outport  Port=2
  adlocb_out : Outport  Port=3
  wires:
  d/1 -> Assert/1
  a/1 -> Assert1/1
  w/1 -> Assert2/1
  r/1 -> Assert4/1
  be/1 -> Assert3/1
  adlocb_in/1 -> Assert5/1
  Configurable Subsystem/1(q) -> Assert6/1
  Configurable Subsystem/2(qv) -> Assert7/1
  Configurable Subsystem/3(adlocb_out) -> Assert8/1
  Assert/1 -> Configurable Subsystem/1(d)
  Assert1/1 -> Configurable Subsystem/2(a)
  Assert2/1 -> Configurable Subsystem/3(w)
  Assert4/1 -> Configurable Subsystem/4(r)
  Assert3/1 -> Configurable Subsystem/5(be)
  Assert5/1 -> Configurable Subsystem/6(adlocb_in)
  Assert8/1 -> adlocb_out/1
  Assert7/1 -> qv/1
  Assert6/1 -> q/1

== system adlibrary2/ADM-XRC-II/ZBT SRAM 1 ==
  d : Inport
  a : Inport  Port=2
  w : Inport  Port=3
  r : Inport  Port=4
  be : Inport  Port=5
  adlocb_in : Inport  Port=6
  Assert{,1..8} (9 alike) : xbsIndex_r4/Assert  assert_type=off  type_source=Explicitly  arith_type="Signed  (2's comp)"  n_bits=16  bin_pt=14  assert_rate=on  rate_source=Explicitly  period=ad_get_simulink_period  output_port=on  block_type=assert
  Configurable Subsystem : Subsystem  Tag=configX  BlockChoice=ZBT SRAM 32Bit Simulation
  q : Outport
  qv : Outport  Port=2
  adlocb_out : Outport  Port=3
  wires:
  Configurable Subsystem/3(adlocb_out) -> Assert8/1
  Configurable Subsystem/2(qv) -> Assert7/1
  Configurable Subsystem/1(q) -> Assert6/1
  adlocb_in/1 -> Assert5/1
  be/1 -> Assert4/1
  r/1 -> Assert3/1
  w/1 -> Assert2/1
  a/1 -> Assert1/1
  d/1 -> Assert/1
  Assert/1 -> Configurable Subsystem/1(d)
  Assert1/1 -> Configurable Subsystem/2(a)
  Assert2/1 -> Configurable Subsystem/3(w)
  Assert3/1 -> Configurable Subsystem/4(r)
  Assert4/1 -> Configurable Subsystem/5(be)
  Assert5/1 -> Configurable Subsystem/6(adlocb_in)
  Assert6/1 -> q/1
  Assert7/1 -> qv/1
  Assert8/1 -> adlocb_out/1

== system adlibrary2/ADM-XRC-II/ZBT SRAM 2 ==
  d : Inport
  a : Inport  Port=2
  w : Inport  Port=3
  r : Inport  Port=4
  be : Inport  Port=5
  adlocb_in : Inport  Port=6
  Assert{,1..8} (9 alike) : xbsIndex_r4/Assert  assert_type=off  type_source=Explicitly  arith_type="Signed  (2's comp)"  n_bits=16  bin_pt=14  assert_rate=on  rate_source=Explicitly  period=ad_get_simulink_period  output_port=on  block_type=assert
  Configurable Subsystem : Subsystem  Tag=configX  BlockChoice=ZBT SRAM 32Bit Simulation
  q : Outport
  qv : Outport  Port=2
  adlocb_out : Outport  Port=3
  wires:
  Configurable Subsystem/3(adlocb_out) -> Assert8/1
  Configurable Subsystem/2(qv) -> Assert7/1
  Configurable Subsystem/1(q) -> Assert6/1
  adlocb_in/1 -> Assert5/1
  be/1 -> Assert4/1
  r/1 -> Assert3/1
  w/1 -> Assert2/1
  a/1 -> Assert1/1
  d/1 -> Assert/1
  Assert/1 -> Configurable Subsystem/1(d)
  Assert1/1 -> Configurable Subsystem/2(a)
  Assert2/1 -> Configurable Subsystem/3(w)
  Assert3/1 -> Configurable Subsystem/4(r)
  Assert4/1 -> Configurable Subsystem/5(be)
  Assert5/1 -> Configurable Subsystem/6(adlocb_in)
  Assert6/1 -> q/1
  Assert7/1 -> qv/1
  Assert8/1 -> adlocb_out/1

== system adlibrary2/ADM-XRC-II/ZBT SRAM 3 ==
  d : Inport
  a : Inport  Port=2
  w : Inport  Port=3
  r : Inport  Port=4
  be : Inport  Port=5
  adlocb_in : Inport  Port=6
  Assert{,1..8} (9 alike) : xbsIndex_r4/Assert  assert_type=off  type_source=Explicitly  arith_type="Signed  (2's comp)"  n_bits=16  bin_pt=14  assert_rate=on  rate_source=Explicitly  period=ad_get_simulink_period  output_port=on  block_type=assert
  Configurable Subsystem : Subsystem  Tag=configX  BlockChoice=ZBT SRAM 32Bit Simulation
  q : Outport
  qv : Outport  Port=2
  adlocb_out : Outport  Port=3
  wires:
  Configurable Subsystem/3(adlocb_out) -> Assert7/1
  Configurable Subsystem/2(qv) -> Assert6/1
  Configurable Subsystem/1(q) -> Assert8/1
  adlocb_in/1 -> Assert5/1
  be/1 -> Assert4/1
  r/1 -> Assert3/1
  w/1 -> Assert2/1
  a/1 -> Assert1/1
  d/1 -> Assert/1
  Assert/1 -> Configurable Subsystem/1(d)
  Assert1/1 -> Configurable Subsystem/2(a)
  Assert2/1 -> Configurable Subsystem/3(w)
  Assert3/1 -> Configurable Subsystem/4(r)
  Assert4/1 -> Configurable Subsystem/5(be)
  Assert5/1 -> Configurable Subsystem/6(adlocb_in)
  Assert8/1 -> q/1
  Assert6/1 -> qv/1
  ? -> adlocb_out/1

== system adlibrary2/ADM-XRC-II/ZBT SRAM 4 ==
  d : Inport
  a : Inport  Port=2
  w : Inport  Port=3
  r : Inport  Port=4
  be : Inport  Port=5
  adlocb_in : Inport  Port=6
  Assert{,1..8} (9 alike) : xbsIndex_r4/Assert  assert_type=off  type_source=Explicitly  arith_type="Signed  (2's comp)"  n_bits=16  bin_pt=14  assert_rate=on  rate_source=Explicitly  period=ad_get_simulink_period  output_port=on  block_type=assert
  Configurable Subsystem : Subsystem  Tag=configX  BlockChoice=ZBT SRAM 32Bit Simulation
  q : Outport
  qv : Outport  Port=2
  adlocb_out : Outport  Port=3
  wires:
  Configurable Subsystem/3(adlocb_out) -> Assert8/1
  Configurable Subsystem/2(qv) -> Assert7/1
  Configurable Subsystem/1(q) -> Assert6/1
  adlocb_in/1 -> Assert5/1
  be/1 -> Assert4/1
  r/1 -> Assert3/1
  w/1 -> Assert2/1
  a/1 -> Assert1/1
  d/1 -> Assert/1
  Assert/1 -> Configurable Subsystem/1(d)
  Assert1/1 -> Configurable Subsystem/2(a)
  Assert2/1 -> Configurable Subsystem/3(w)
  Assert3/1 -> Configurable Subsystem/4(r)
  Assert4/1 -> Configurable Subsystem/5(be)
  Assert5/1 -> Configurable Subsystem/6(adlocb_in)
  Assert6/1 -> q/1
  Assert7/1 -> qv/1
  Assert8/1 -> adlocb_out/1

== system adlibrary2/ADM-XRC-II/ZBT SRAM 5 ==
  d : Inport
  a : Inport  Port=2
  w : Inport  Port=3
  r : Inport  Port=4
  be : Inport  Port=5
  adlocb_in : Inport  Port=6
  Assert{,1..8} (9 alike) : xbsIndex_r4/Assert  assert_type=off  type_source=Explicitly  arith_type="Signed  (2's comp)"  n_bits=16  bin_pt=14  assert_rate=on  rate_source=Explicitly  period=ad_get_simulink_period  output_port=on  block_type=assert
  Configurable Subsystem : Subsystem  Tag=configX  BlockChoice=ZBT SRAM 32Bit Simulation
  q : Outport
  qv : Outport  Port=2
  adlocb_out : Outport  Port=3
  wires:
  Configurable Subsystem/3(adlocb_out) -> Assert8/1
  Configurable Subsystem/2(qv) -> Assert7/1
  Configurable Subsystem/1(q) -> Assert6/1
  adlocb_in/1 -> Assert5/1
  be/1 -> Assert4/1
  r/1 -> Assert3/1
  w/1 -> Assert2/1
  a/1 -> Assert1/1
  d/1 -> Assert/1
  Assert/1 -> Configurable Subsystem/1(d)
  Assert1/1 -> Configurable Subsystem/2(a)
  Assert2/1 -> Configurable Subsystem/3(w)
  Assert3/1 -> Configurable Subsystem/4(r)
  Assert4/1 -> Configurable Subsystem/5(be)
  Assert5/1 -> Configurable Subsystem/6(adlocb_in)
  Assert6/1 -> q/1
  Assert7/1 -> qv/1
  Assert8/1 -> adlocb_out/1

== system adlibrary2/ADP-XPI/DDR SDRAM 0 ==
  cache_data_in : Inport
  cache_addr : Inport  Port=2
  cache_write : Inport  Port=3
  ddr_page : Inport  Port=4
  ddr_addr : Inport  Port=5
  ddr_read : Inport  Port=6
  ddr_write : Inport  Port=7
  Assert{1..7,9..10} (9 alike) : xbsIndex_r4/Assert  assert_type=off  type_source=Explicitly  arith_type="Signed  (2's comp)"  n_bits=16  bin_pt=14  assert_rate=on  rate_source=Explicitly  period=ad_get_simulink_period  output_port=on  block_type=assert
  Configurable Subsystem : Subsystem  Tag=configX  BlockChoice=DDR SDRAM 64bit Simulation  mask{memsize=memsize}
      mask prompts: memsize "Simulation Ram Size (Mb)"
  cache_data_out : Outport
  ddr_busy : Outport  Port=2
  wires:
  Assert10/1 -> ddr_busy/1
  Assert9/1 -> cache_data_out/1
  Assert6/1 -> Configurable Subsystem/6(ddr_read)
  Assert5/1 -> Configurable Subsystem/5(ddr_addr)
  Assert4/1 -> Configurable Subsystem/4(ddr_page)
  Assert3/1 -> Configurable Subsystem/3(cache_write)
  Assert2/1 -> Configurable Subsystem/2(cache_addr)
  Assert1/1 -> Configurable Subsystem/1(cache_data_in)
  ddr_write/1 -> Assert7/1
  ddr_read/1 -> Assert6/1
  ddr_addr/1 -> Assert5/1
  ddr_page/1 -> Assert4/1
  cache_write/1 -> Assert3/1
  cache_addr/1 -> Assert2/1
  cache_data_in/1 -> Assert1/1
  Configurable Subsystem/1(cache_data_out) -> Assert9/1
  Configurable Subsystem/2(ddr_busy) -> Assert10/1
  Assert7/1 -> Configurable Subsystem/7(ddr_write)

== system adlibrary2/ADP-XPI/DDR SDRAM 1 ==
  cache_data_in : Inport
  cache_addr : Inport  Port=2
  cache_write : Inport  Port=3
  ddr_page : Inport  Port=4
  ddr_addr : Inport  Port=5
  ddr_read : Inport  Port=6
  ddr_write : Inport  Port=7
  Assert{1..7,9..10} (9 alike) : xbsIndex_r4/Assert  assert_type=off  type_source=Explicitly  arith_type="Signed  (2's comp)"  n_bits=16  bin_pt=14  assert_rate=on  rate_source=Explicitly  period=ad_get_simulink_period  output_port=on  block_type=assert
  Configurable Subsystem : Subsystem  Tag=configX  BlockChoice=DDR SDRAM 64bit Simulation  mask{memsize=memsize}
      mask prompts: memsize "Simulation Ram Size (Mb)"
  cache_data_out : Outport
  ddr_busy : Outport  Port=2
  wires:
  Assert7/1 -> Configurable Subsystem/7(ddr_write)
  Configurable Subsystem/2(ddr_busy) -> Assert10/1
  Configurable Subsystem/1(cache_data_out) -> Assert9/1
  cache_data_in/1 -> Assert1/1
  cache_addr/1 -> Assert2/1
  cache_write/1 -> Assert3/1
  ddr_page/1 -> Assert4/1
  ddr_addr/1 -> Assert5/1
  ddr_read/1 -> Assert6/1
  ddr_write/1 -> Assert7/1
  Assert1/1 -> Configurable Subsystem/1(cache_data_in)
  Assert2/1 -> Configurable Subsystem/2(cache_addr)
  Assert3/1 -> Configurable Subsystem/3(cache_write)
  Assert4/1 -> Configurable Subsystem/4(ddr_page)
  Assert5/1 -> Configurable Subsystem/5(ddr_addr)
  Assert6/1 -> Configurable Subsystem/6(ddr_read)
  Assert9/1 -> cache_data_out/1
  Assert10/1 -> ddr_busy/1

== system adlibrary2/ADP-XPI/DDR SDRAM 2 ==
  cache_data_in : Inport
  cache_addr : Inport  Port=2
  cache_write : Inport  Port=3
  ddr_page : Inport  Port=4
  ddr_addr : Inport  Port=5
  ddr_read : Inport  Port=6
  ddr_write : Inport  Port=7
  Assert{1..7,9..10} (9 alike) : xbsIndex_r4/Assert  assert_type=off  type_source=Explicitly  arith_type="Signed  (2's comp)"  n_bits=16  bin_pt=14  assert_rate=on  rate_source=Explicitly  period=ad_get_simulink_period  output_port=on  block_type=assert
  Configurable Subsystem : Subsystem  Tag=configX  BlockChoice=DDR SDRAM 64bit Simulation  mask{memsize=memsize}
      mask prompts: memsize "Simulation Ram Size (Mb)"
  cache_data_out : Outport
  ddr_busy : Outport  Port=2
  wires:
  Assert10/1 -> ddr_busy/1
  Assert9/1 -> cache_data_out/1
  Assert6/1 -> Configurable Subsystem/6(ddr_read)
  Assert5/1 -> Configurable Subsystem/5(ddr_addr)
  Assert4/1 -> Configurable Subsystem/4(ddr_page)
  Assert3/1 -> Configurable Subsystem/3(cache_write)
  Assert2/1 -> Configurable Subsystem/2(cache_addr)
  Assert1/1 -> Configurable Subsystem/1(cache_data_in)
  ddr_write/1 -> Assert7/1
  ddr_read/1 -> Assert6/1
  ddr_addr/1 -> Assert5/1
  ddr_page/1 -> Assert4/1
  cache_write/1 -> Assert3/1
  cache_addr/1 -> Assert2/1
  cache_data_in/1 -> Assert1/1
  Configurable Subsystem/1(cache_data_out) -> Assert9/1
  Configurable Subsystem/2(ddr_busy) -> Assert10/1
  Assert7/1 -> Configurable Subsystem/7(ddr_write)

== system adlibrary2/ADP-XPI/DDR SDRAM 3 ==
  cache_data_in : Inport
  cache_addr : Inport  Port=2
  cache_write : Inport  Port=3
  ddr_page : Inport  Port=4
  ddr_addr : Inport  Port=5
  ddr_read : Inport  Port=6
  ddr_write : Inport  Port=7
  Assert{1..7,9..10} (9 alike) : xbsIndex_r4/Assert  assert_type=off  type_source=Explicitly  arith_type="Signed  (2's comp)"  n_bits=16  bin_pt=14  assert_rate=on  rate_source=Explicitly  period=ad_get_simulink_period  output_port=on  block_type=assert
  Configurable Subsystem : Subsystem  Tag=configX  BlockChoice=DDR SDRAM 64bit Simulation  mask{memsize=memsize}
      mask prompts: memsize "Simulation Ram Size (Mb)"
  cache_data_out : Outport
  ddr_busy : Outport  Port=2
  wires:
  Assert7/1 -> Configurable Subsystem/7(ddr_write)
  Configurable Subsystem/2(ddr_busy) -> Assert10/1
  Configurable Subsystem/1(cache_data_out) -> Assert9/1
  cache_data_in/1 -> Assert1/1
  cache_addr/1 -> Assert2/1
  cache_write/1 -> Assert3/1
  ddr_page/1 -> Assert4/1
  ddr_addr/1 -> Assert5/1
  ddr_read/1 -> Assert6/1
  ddr_write/1 -> Assert7/1
  Assert1/1 -> Configurable Subsystem/1(cache_data_in)
  Assert2/1 -> Configurable Subsystem/2(cache_addr)
  Assert3/1 -> Configurable Subsystem/3(cache_write)
  Assert4/1 -> Configurable Subsystem/4(ddr_page)
  Assert5/1 -> Configurable Subsystem/5(ddr_addr)
  Assert6/1 -> Configurable Subsystem/6(ddr_read)
  Assert9/1 -> cache_data_out/1
  Assert10/1 -> ddr_busy/1
